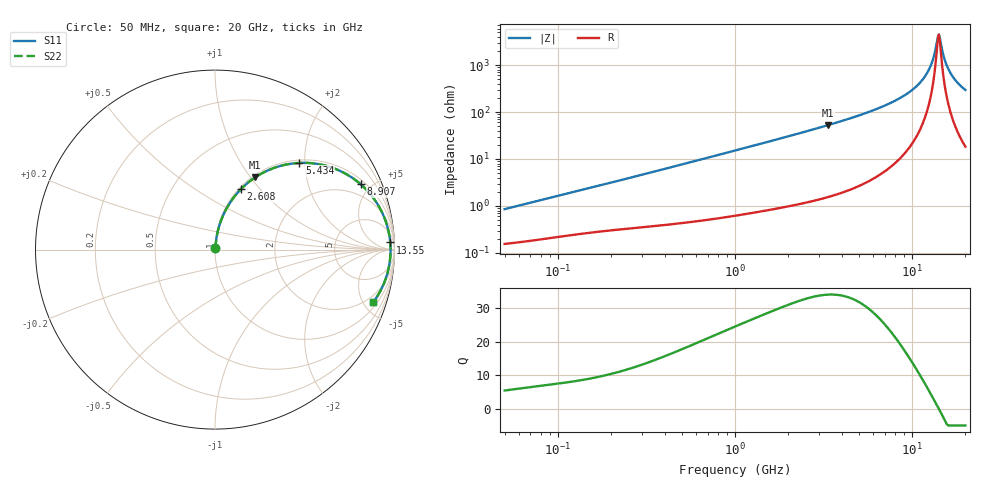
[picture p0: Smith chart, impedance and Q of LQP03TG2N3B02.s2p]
!Murata Part Number: LQP03TG2N3B02
!These Parameters are Measured in Series Mode Connection
!  o--[Z]--o
!Port1  Port2
!  o-------o
!Freq. Start=50[MHz] Stop=20[GHz], 401[Steps]
# Hz S RI R 50
!Freq.(Hz) S11(Real) S11(Imag) S21(Real) S21(Imag) S12(Real) S12(Imag) S22(Real) S22(Imag)
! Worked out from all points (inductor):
!   401 points, 50 MHz to 20 GHz, reference 50 ohm
!   read as one part in series: L = 2.65 nH near 51.52 MHz
!   highest Q = 34 at 3.364 GHz (marker M1), where L = 2.5 nH
!   self-resonance near 13.96 GHz
!   S11 on the Smith chart (normalised r, x): 50 MHz: 1.00, +0.02; 2.608 GHz: 1.02, +0.80; 5.434 GHz: 1.06, +1.88; 8.907 GHz: 1.24, +4.34; 13.55 GHz: 21, +37; 20 GHz: 1.37, -5.88
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5e7  0.00162 0.00839  0.9984 -0.00839  0.9984 -0.00839  0.00162 0.00839
1.364002e8  0.00303 0.0217  0.997 -0.0217  0.997 -0.0217  0.00303 0.0217
3.721004e8  0.00702 0.0565  0.993 -0.0565  0.993 -0.0565  0.00702 0.0565
1e9  0.0281 0.146  0.9719 -0.146  0.9719 -0.146  0.0281 0.146
2.608132e9  0.1456 0.3379  0.8544 -0.3379  0.8544 -0.3379  0.1456 0.3379
2.728004e9  0.1574 0.3494  0.8426 -0.3494  0.8426 -0.3494  0.1574 0.3494
3.364474e9  0.2245 0.4028  0.7755 -0.4028  0.7755 -0.4028  0.2245 0.4028
5.433528e9  0.4702 0.483  0.5298 -0.483  0.5298 -0.483  0.4702 0.483
7.442007e9  0.6894 0.4419  0.3106 -0.4419  0.3106 -0.4419  0.6894 0.4419
8.907419e9  0.8119 0.3638  0.1881 -0.3638  0.1881 -0.3638  0.8119 0.3638
1.050288e10  0.904 0.2559  0.096 -0.2559  0.096 -0.2559  0.904 0.2559
1.183995e10  0.9505 0.1595  0.0495 -0.1595  0.0495 -0.1595  0.9505 0.1595
1.276073e10  0.9686 0.0938  0.0314 -0.0938  0.0314 -0.0938  0.9686 0.0938
1.314879e10  0.9733 0.0668  0.0267 -0.0668  0.0267 -0.0668  0.9733 0.0668
1.354865e10  0.9764 0.0396  0.0236 -0.0396  0.0236 -0.0396  0.9764 0.0396
1.396067e10  0.978 0.0121  0.022 -0.0121  0.022 -0.0121  0.978 0.0121
1.417136e10  0.9782 -0.00163  0.0218 0.00163  0.0218 0.00163  0.9782 -0.00163
1.438523e10  0.978 -0.0154  0.022 0.0154  0.022 0.0154  0.978 -0.0154
1.527346e10  0.9735 -0.0701  0.0265 0.0701  0.0265 0.0701  0.9735 -0.0701
1.621653e10  0.9628 -0.1239  0.0372 0.1239  0.0372 0.1239  0.9628 -0.1239
1.774144e10  0.9359 -0.2008  0.0641 0.2008  0.0641 0.2008  0.9359 -0.2008
2e10  0.8821 -0.2929  0.1179 0.2929  0.1179 0.2929  0.8821 -0.2929
